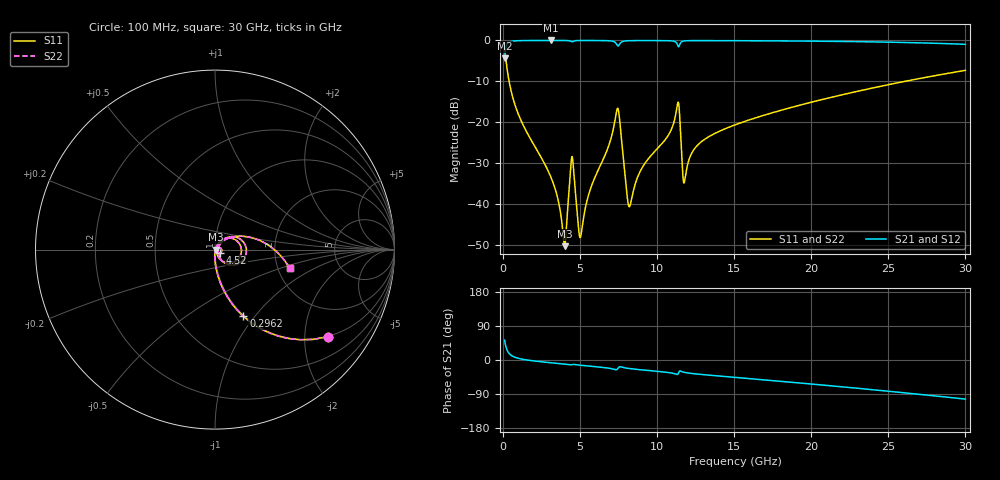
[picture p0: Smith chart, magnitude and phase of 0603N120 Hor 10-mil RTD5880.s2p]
# GHz S MA R 50
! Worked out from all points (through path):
!   3201 points, 100 MHz to 30 GHz, reference 50 ohm
!   highest |S21| = -0.02 dB at 3.109 GHz (marker M1); lowest = -4.3 dB at 100 MHz (marker M2)
!   group delay of S21, straight-line fit = 9.92 ps
!   lowest |S11| = -50.3 dB at 3.996 GHz (marker M3), VSWR 1.01, Z = 50.3 - j0.111 ohm
!   |S11| at or under -10 dB: 390.6 MHz to 26.1 GHz (25.71 GHz wide, 194 % of centre)
!   |S22| runs from -50.3 to -2.0 dB; largest |S21 - S12| = 0
!   S11 on the Smith chart (normalised r, x): 100 MHz: 0.99, -2.61; 296.2 MHz: 0.99, -0.88; 4.52 GHz: 1.06, -0.04; 30 GHz: 2.32, -0.60
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0.1  0.7951 -37.6  0.6062 52.4  0.6062 52.4  0.7951 -37.6
0.2962187  0.4034 -67.0  0.9145 23.0  0.9145 23.0  0.4034 -67.0
1.043719  0.1183 -85.6  0.9921 3.9  0.9921 3.9  0.1183 -85.6
3.108687  0.02113 -92.8  0.9981 -7.3  0.9981 -7.3  0.02113 -92.8
3.996344  0.003039 -21.4  0.997 -10.9  0.997 -10.9  0.003039 -21.4
4.379437  0.02655 27.7  0.9797 -13.0  0.9797 -13.0  0.02655 27.7
4.519594  0.03453 -32.9  0.9677 -11.7  0.9677 -11.7  0.03453 -32.9
4.902687  0.004927 -39.2  0.9955 -13.3  0.9955 -13.3  0.004927 -39.2
5.089563  0.004544 25.7  0.9964 -14.1  0.9964 -14.1  0.004544 25.7
5.594125  0.01377 61.1  0.9968 -16.1  0.9968 -16.1  0.01377 61.1
7.397469  0.1435 8.9  0.8773 -24.8  0.8773 -24.8  0.1435 8.9
7.556312  0.1106 -42.8  0.8984 -18.0  0.8984 -18.0  0.1106 -42.8
8.191688  0.009211 -4.8  0.9911 -22.5  0.9911 -22.5  0.009211 -4.8
8.939187  0.02589 53.5  0.9948 -25.8  0.9948 -25.8  0.02589 53.5
10.06978  0.04871 54.5  0.9942 -30.2  0.9942 -30.2  0.04871 54.5
11.33119  0.1706 8.3  0.8741 -37.9  0.8741 -37.9  0.1706 8.3
11.78903  0.01949 15.0  0.9866 -32.8  0.9866 -32.8  0.01949 15.0
12.62997  0.05252 47.7  0.9938 -37.2  0.9938 -37.2  0.05252 47.7
15.05  0.09257 41.6  0.9915 -45.9  0.9915 -45.9  0.09257 41.6
20.03956  0.176 24.9  0.9793 -63.5  0.9793 -63.5  0.176 24.9
25.01978  0.2877 6.3  0.9516 -82.5  0.9516 -82.5  0.2877 6.3
30  0.43 -14.1  0.8954 -103.2  0.8954 -103.2  0.43 -14.1
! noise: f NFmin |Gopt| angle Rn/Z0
0.1  0.0003162  0.9246  0.5067  0.0009287
3.417  0.003712  0.795  9.399  0.003718
6.743  0.01008  0.8474  18.41  0.01369
10.06  0.009928  0.7788  27.3  0.008689
13.39  0.01094  0.7408  36.05  0.007665
16.7  0.01242  0.7213  44.5  0.007599
20.03  0.01447  0.7173  52.8  0.008174
23.35  0.01672  0.7181  60.85  0.008807
26.67  0.0192  0.7225  68.71  0.009465
30  0.02196  0.7296  76.35  0.01015
